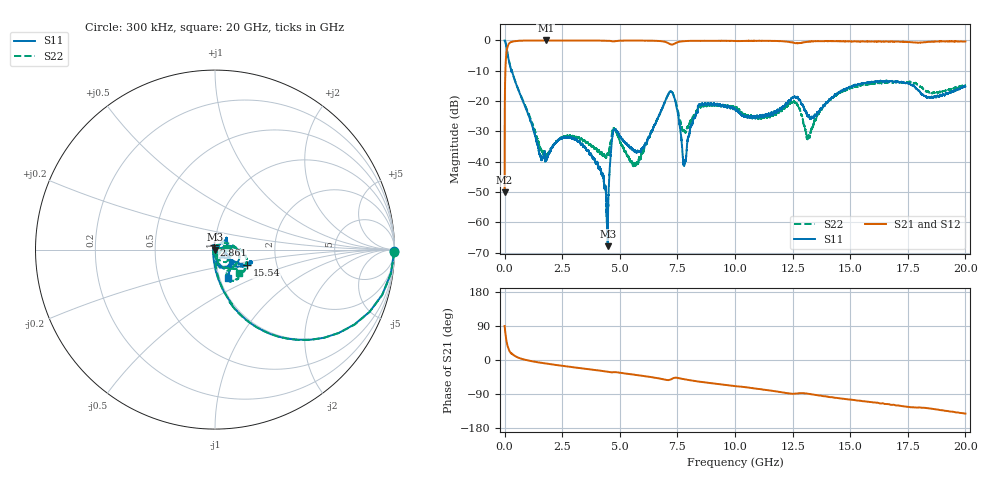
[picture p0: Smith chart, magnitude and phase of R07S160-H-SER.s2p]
!{R07S160}
!Johanson Technology Inc.
!www.johansontechnology.com
!Test Board Conditions:
!Substrate Type  RO4350B
!Substrate Thickness  10 mil
!Substrate Dk  3.66
!TL Type: GCPW
!TL Trace Width  21 mil
!TL Gap  20 mil
!Electrode orientation  Horizontal
!DUT TOPOLOGY	SERIES
!Mounting Pad LxW  16x21 mil
! Created Sat Feb  6 11:48:00 2021
# hz S ma R 50
! 2 Port Network Data from SP1.SP block
! freq  magS11  angS11  magS21  angS21  magS12  angS12  magS22  angS22
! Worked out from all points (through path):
!   20001 points, 300 kHz to 20 GHz, reference 50 ohm
!   highest |S21| = -0.01 dB at 1.784 GHz (marker M1); lowest = -50.1 dB at 300 kHz (marker M2)
!   group delay of S21, straight-line fit = 20.5 ps
!   lowest |S11| = -67.8 dB at 4.473 GHz (marker M3), VSWR 1.00, Z = 50 - j0.0169 ohm
!   |S11| at or under -10 dB: 286.1 MHz to 299.8 MHz (13.74 MHz wide, 4.69 % of centre); 313.6 MHz to end of sweep
!   |S22| runs from -41.5 to 0.0 dB; largest |S21 - S12| = 0.014
!   S11 on the Smith chart (normalised r, x): 300 kHz: open; 2.861 GHz: 0.98, +0.05; 15.54 GHz: 1.40, -0.25; 20 GHz: 1.10, -0.36
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300000  0.9984 -0.5  0.003135 89.6  0.003103 88.1  1 -0.7
1.033e8  0.6872 -47.0  0.7216 43.3  0.7233 43.2  0.688 -47.0
1.833e8  0.4686 -63.3  0.8787 27.2  0.8797 27.3  0.4678 -63.3
1.7843e9  0.01058 159.6  0.9984 -9.3  0.9972 -9.3  0.01233 -16.9
2.8613e9  0.02514 108.8  0.9961 -18.1  0.9967 -18.2  0.02673 20.8
3.3343e9  0.01957 114.2  0.9956 -21.9  0.9965 -21.8  0.02401 6.5
4.1913e9  0.006839 170.1  0.9938 -28.6  0.9945 -28.6  0.01447 -33.7
4.4733e9  0.0004059 -24.6  0.9906 -31.0  0.9899 -31.0  0.01355 -23.9
4.7663e9  0.03354 -73.4  0.9692 -31.9  0.9692 -32.0  0.03467 -65.7
5.6723e9  0.01494 -66.2  0.9955 -39.2  0.996 -39.2  0.009108 155.1
6.6673e9  0.05428 17.8  0.9817 -48.2  0.9823 -48.2  0.05299 39.9
7.2813e9  0.1391 -43.4  0.8557 -49.2  0.8568 -49.1  0.1391 -42.9
7.8073e9  0.00972 -6.5  0.9772 -50.9  0.9769 -50.9  0.03174 -35.1
8.4873e9  0.08664 44.4  0.985 -57.4  0.9851 -57.4  0.07898 16.2
1.00003e10  0.07437 24.0  0.9793 -69.0  0.9804 -69.0  0.07721 -2.4
1.25753e10  0.1186 -51.4  0.9105 -88.9  0.9112 -89.0  0.09694 -36.9
1.33343e10  0.05428 -60.9  0.9649 -90.5  0.9664 -90.6  0.03573 2.4
1.41473e10  0.1074 -32.8  0.9746 -98.1  0.9757 -98.0  0.1047 7.0
1.55383e10  0.1971 -26.0  0.9671 -108.5  0.9621 -108.3  0.1851 -16.9
1.66673e10  0.2085 -19.2  0.9503 -116.6  0.9574 -117.0  0.2049 -39.9
1.84073e10  0.1168 -36.2  0.9496 -127.4  0.949 -127.1  0.1414 -60.4
2e10  0.1753 -65.3  0.9632 -141.6  0.9557 -141.5  0.1842 -44.9
